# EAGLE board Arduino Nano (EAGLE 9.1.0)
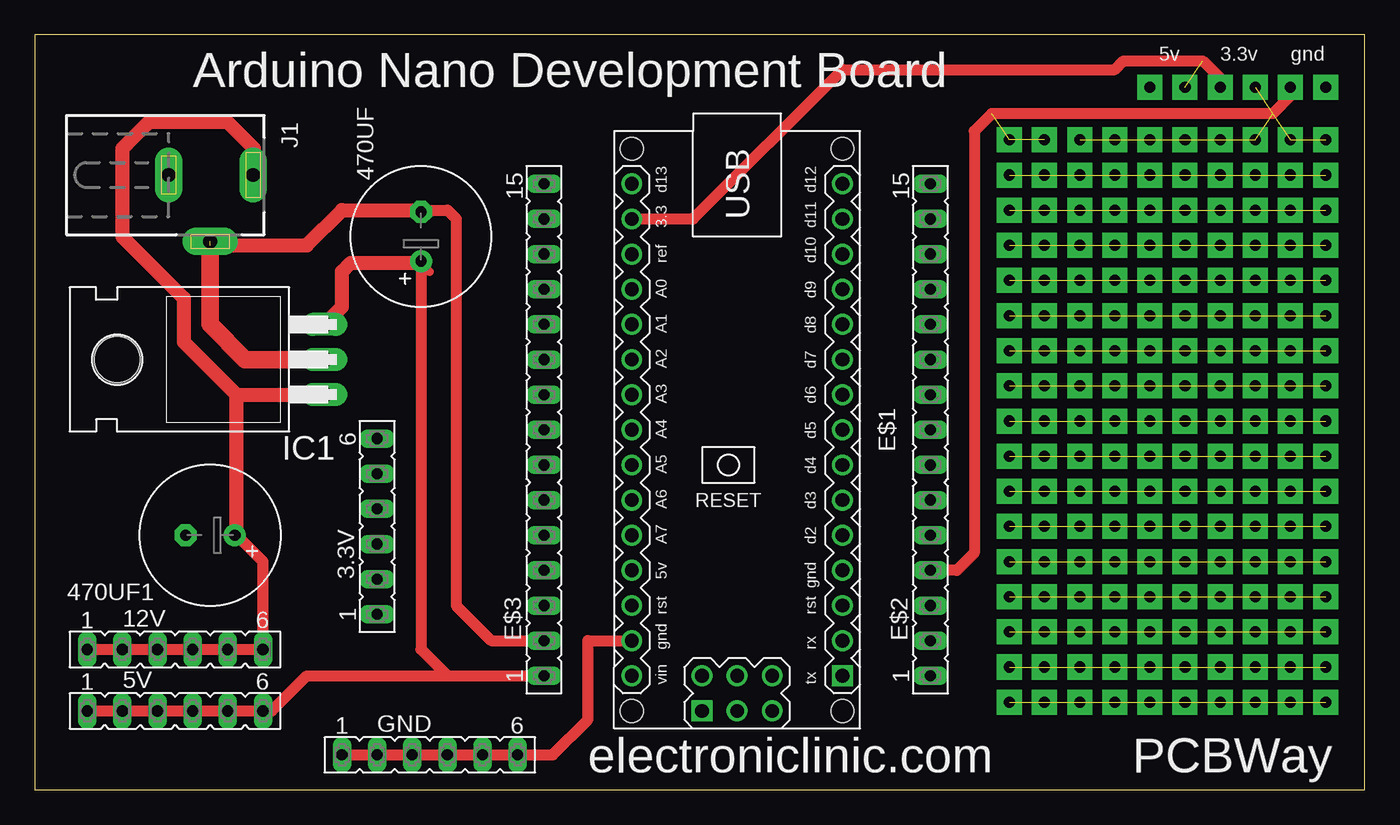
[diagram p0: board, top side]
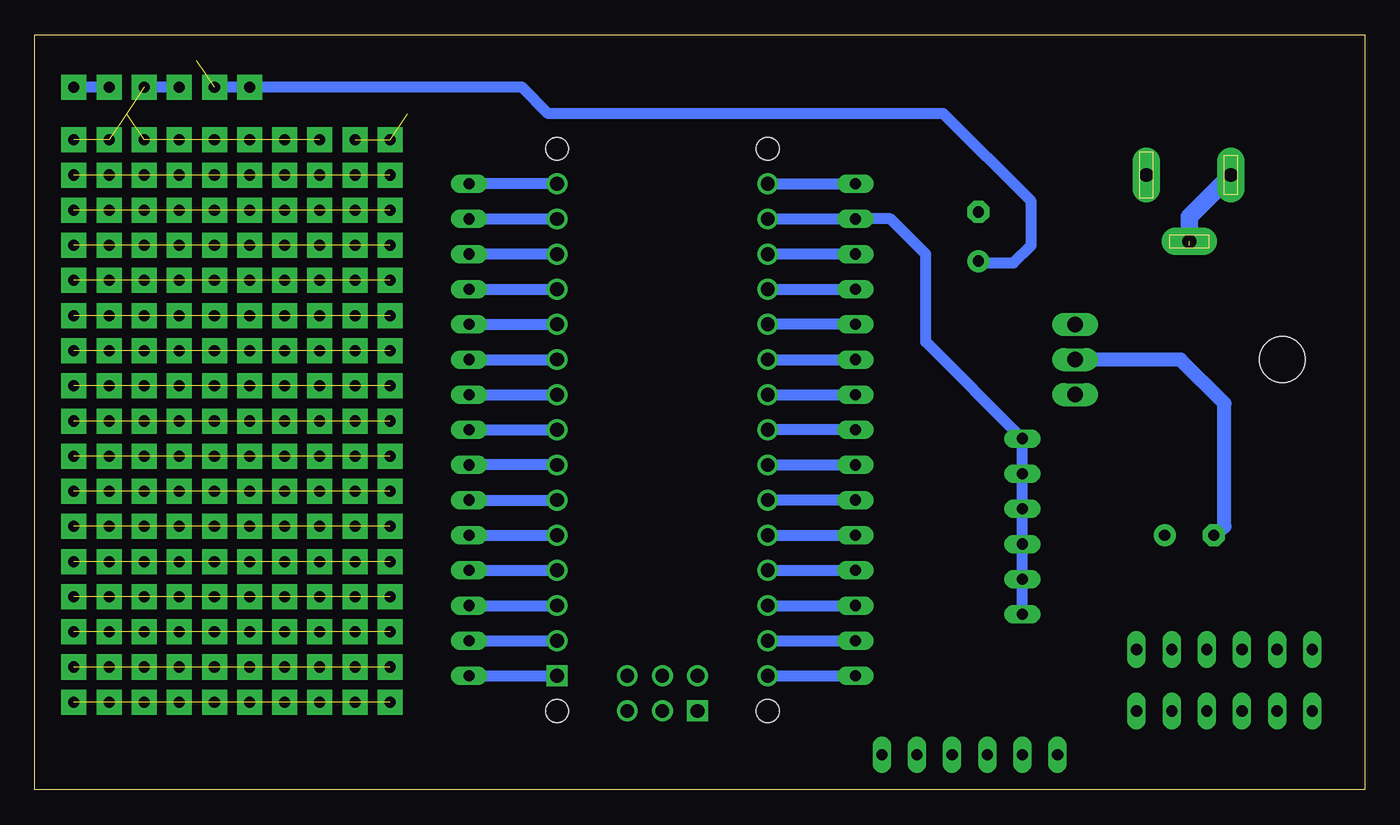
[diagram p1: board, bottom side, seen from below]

Size 96.19 x 54.6 mm. Coordinates in mm from the lower left corner, seen from the top.
Outline: 0,0 96.19,0 96.19,54.6 0,54.6 0,0
Copper layers (1*16): Top 0.035mm / dielectric 1.5mm / Bottom 0.035mm
Design rules "default": minimum track width 6mil, minimum drill 0.35mm, track to track 6mil, track to pad 6mil, pad to pad 6mil, via to via 6mil, smd to smd 6mil, copper to edge 40mil, drill to drill 6mil, minimum pad ring 10mil, minimum via ring 8mil, stop-mask expansion 4mil, vias tented up to drill 0mil, thermal gap 10mil

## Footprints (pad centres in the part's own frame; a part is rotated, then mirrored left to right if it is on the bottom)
FE06 = drill 0.813 long: 1 -6.35,0; 2 -3.81,0; 3 -1.27,0; 4 1.27,0; 5 3.81,0; 6 6.35,0
E3,5-10 = drill 0.813 pad 1.6: + -1.778,0 | drill 0.813 pad 1.6 octagon: - 1.778,0
ARDUINO-NANO-3.0#ISP = drill 1 square: J1.1 17.78,7.62; J4.1 20.32,-2.54 | drill 1: J1.2 15.24,7.62; J1.3 12.7,7.62; J1.4 10.16,7.62; J1.5 7.62,7.62; J1.6 5.08,7.62; J1.7 2.54,7.62; J1.8 0,7.62; J1.9 -2.54,7.62; J1.10 -5.08,7.62; J1.11 -7.62,7.62; J1.12 -10.16,7.62; J1.13 -12.7,7.62; J1.14 -15.24,7.62; J1.15 -17.78,7.62; J2.1 17.78,-7.62; J2.2 15.24,-7.62; J2.3 12.7,-7.62; J2.4 10.16,-7.62; J2.5 7.62,-7.62; J2.6 5.08,-7.62; J2.7 2.54,-7.62; J2.8 0,-7.62; J2.9 -2.54,-7.62; J2.10 -5.08,-7.62; J2.11 -7.62,-7.62; J2.12 -10.16,-7.62; J2.13 -12.7,-7.62; J2.14 -15.24,-7.62; J2.15 -17.78,-7.62; J4.2 17.78,-2.54; J4.3 20.32,0; J4.4 17.78,0; J4.5 20.32,2.54; J4.6 17.78,2.54 | hole 1.651: -20.32,7.62; -20.32,-7.62; 20.32,-7.62; 20.32,7.62
FE15 = drill 0.813 long: 1 -17.78,0; 2 -15.24,0; 3 -12.7,0; 4 -10.16,0; 5 -7.62,0; 6 -5.08,0; 7 -2.54,0; 8 0,0; 9 2.54,0; 10 5.08,0; 11 7.62,0; 12 10.16,0; 13 12.7,0; 14 15.24,0; 15 17.78,0
TO220H = drill 1.118 long: 1 -2.54,-10.16; 2 0,-10.16; 3 2.54,-10.16 | hole 3.302: 0,4.826
DCJ0202 = drill 1 pad 2 long: 1 0,3.1; 2 4.8,0; 3 0,-3

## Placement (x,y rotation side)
3.3V  [FE06]  24.77,19.05 90 top
5V  [FE06]  10.16,5.71 0 top
12V  [FE06]  10.16,10.16 0 top
470UF  [E3,5-10]  27.94,40.01 90 top
470UF1  [E3,5-10]  12.7,18.41 180 top
E$1  [ARDUINO-NANO-3.0#ISP]  50.8,26.04 270 top
E$2  [FE15]  64.77,26.04 90 top
E$3  [FE15]  36.83,26.04 90 top
GND  [FE06]  28.57,2.54 0 top
IC1  7805T  [TO220H]  10.79,31.11 90 top
J1  DCJ0202  [DCJ0202]  12.7,44.45 270 top

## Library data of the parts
3.3V 5V 12V E$2 E$3 GND = con-lsta
470UF 470UF1 = rcl
E$1 = diy-modules
IC1 = linear
J1 = con-jack; OC_FARNELL: unknown; OC_NEWARK: unknown

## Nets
5V: 5V.1 5V.2 5V.3 5V.4 5V.5 5V.6 E$1.J2.1 E$3.1 IC1.3
12V: 12V.1 12V.2 12V.3 12V.4 12V.5 12V.6 IC1.1
GND: E$1.J2.2 E$3.2 GND.1 GND.2 GND.4 GND.5 GND.6 IC1.2 J1.2 J1.3
S$2: E$1.J1.7 E$2.7
S$4: E$1.J1.15 E$2.15
S$5: E$1.J2.4 E$3.4
S$6: E$1.J1.14 E$2.14
S$7: E$1.J2.3 E$3.3
S$8: E$1.J1.13 E$2.13
S$9: E$1.J1.10 E$2.10
S$10: E$1.J1.12 E$2.12
S$11: 3.3V.1 3.3V.2 3.3V.3 3.3V.4 3.3V.5 3.3V.6 E$1.J1.4 E$1.J2.14 E$2.4 E$3.14
S$15: E$1.J1.9 E$2.9
S$16: E$1.J1.8 E$2.8
S$18: E$1.J1.3 E$2.3
S$19: E$1.J1.2 E$2.2
S$20: E$1.J1.1 E$2.1
S$21: E$1.J2.15 E$3.15
S$23: E$1.J2.13 E$3.13
S$24: E$1.J2.12 E$3.12
S$25: E$1.J2.11 E$3.11
S$26: E$1.J2.10 E$3.10
S$27: E$1.J2.9 E$3.9
S$28: E$1.J2.8 E$3.8
S$29: E$1.J2.7 E$3.7
S$30: E$1.J2.6 E$3.6
S$31: E$1.J2.5 E$3.5
S$32: E$1.J1.6 E$2.6
S$34: E$1.J1.5 E$2.5
S$38: E$1.J1.11 E$2.11

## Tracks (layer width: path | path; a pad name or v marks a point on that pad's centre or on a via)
5V
  Top 0.61: 28.57,37.47 27.94,38.1
  Top 0.813: 27.94,38.1 27.94,10.16 29.84,8.26 | 29.84,8.26 30.48,8.26 E$3.1 | 5V.1 5V.2 5V.3 5V.4 5V.5 5V.6 17.14,5.71 19.68,8.26 29.84,8.26
  Top 1.016: IC1.3 22.23,34.92 22.23,37.47 22.86,38.1 27.94,38.1
  Bottom 0.813: E$1.J2.1 E$3.1
12V
  Top 0.813: 12V.1 12V.2 12V.3 12V.4 12V.5 12V.6 16.51,16.51 14.61,18.41
  Top 1.016: 15.88,44.45 15.88,46.35 13.97,48.26 8.26,48.26 6.35,46.35 6.35,40.01 10.79,35.56 10.79,32.38 14.61,28.57 | 14.61,28.57 IC1.1 | 14.61,18.41 14.61,28.57
GND  (1 unrouted)
  Top 0.813: 27.94,41.91 29.84,41.91 30.48,41.27 30.48,13.34 33.02,10.79 E$3.2 | GND.1 GND.2 GND.4 GND.5 GND.6 37.47,2.54 40.01,5.08 40.01,10.79 E$1.J2.2
  Top 1.016: 12.7,39.37 19.68,39.37 22.23,41.91 27.94,41.91
  Top 1.27: 12.7,39.37 12.7,33.66 15.24,31.11 IC1.2
  Bottom 0.813: E$1.J2.2 E$3.2
  Bottom 1.016: 10.79,18.41 10.16,19.05 10.16,27.94 13.34,31.11 IC1.2
  Bottom 1.27: J1.3 12.7,41.45 J1.2
S$2
  Bottom 0.813: E$1.J1.7 E$2.7
S$4
  Bottom 0.813: E$1.J1.15 E$2.15
S$5
  Bottom 0.813: E$1.J2.4 E$3.4
S$6
  Bottom 0.813: E$2.14 E$1.J1.14
S$7
  Bottom 0.813: E$1.J2.3 E$3.3
S$8
  Bottom 0.813: E$1.J1.13 E$2.13
S$9
  Bottom 0.813: E$2.10 E$1.J1.10
S$10
  Bottom 0.813: E$2.12 E$1.J1.12
S$11  (via drill 0.8 pad 1.81)  (12 unrouted)
  Top 0.813: E$1.J2.14 47.62,41.27 58.42,52.07 78.11,52.07 78.74,52.7 84.45,52.7 85.72,51.44 v85.72,50.8 | v90.81,50.8 90.81,50.16 89.53,48.9 69.22,48.9 67.94,47.62 67.94,17.14 66.67,15.88 E$2.4
  Bottom 0.508: 27.94,38.1 26.04,38.1
  Bottom 0.813: 3.3V.1 3.3V.2 3.3V.3 3.3V.4 3.3V.5 3.3V.6 31.75,32.38 31.75,38.73 34.29,41.27 E$3.14 E$1.J2.14 | 27.94,38.1 25.4,38.1 24.13,39.37 24.13,42.55 30.48,48.9 59.05,48.9 60.96,50.8 v80.64,50.8 v83.19,50.8 | v85.72,50.8 v88.27,50.8 | v90.81,50.8 v93.34,50.8 | E$2.4 59.05,15.88 E$1.J1.4
  other vias: 70.48,46.99 73.03,46.99 75.56,46.99 78.11,46.99 80.64,46.99 83.19,46.99 85.72,46.99 88.27,46.99 90.81,46.99 93.34,46.99
S$13  (via drill 0.8 pad 1.81)  (9 unrouted)
  other vias: 70.48,44.45 73.03,44.45 75.56,44.45 78.11,44.45 80.64,44.45 83.19,44.45 85.72,44.45 88.27,44.45 90.81,44.45 93.34,44.45
S$14  (via drill 0.8 pad 1.81)  (9 unrouted)
  other vias: 70.48,41.91 73.03,41.91 75.56,41.91 78.11,41.91 80.64,41.91 83.19,41.91 85.72,41.91 88.27,41.91 90.81,41.91 93.34,41.91
S$15
  Bottom 0.813: E$2.9 E$1.J1.9
S$16
  Bottom 0.813: E$2.8 E$1.J1.8
S$18
  Bottom 0.813: E$2.3 E$1.J1.3
S$19
  Bottom 0.813: E$2.2 E$1.J1.2
S$20
  Bottom 0.813: E$2.1 E$1.J1.1
S$21
  Bottom 0.813: E$1.J2.15 E$3.15
S$22  (via drill 0.8 pad 1.81)  (9 unrouted)
  other vias: 70.48,39.37 73.03,39.37 75.56,39.37 78.11,39.37 80.64,39.37 83.19,39.37 85.72,39.37 88.27,39.37 90.81,39.37 93.34,39.37
S$23
  Bottom 0.813: E$3.13 E$1.J2.13
S$24
  Bottom 0.813: E$1.J2.12 E$3.12
S$25
  Bottom 0.813: E$3.11 E$1.J2.11
S$26
  Bottom 0.813: E$1.J2.10 E$3.10
S$27
  Bottom 0.813: E$1.J2.9 E$3.9
S$28
  Bottom 0.813: E$3.8 E$1.J2.8
S$29
  Bottom 0.813: E$1.J2.7 E$3.7
S$30
  Bottom 0.813: E$3.6 E$1.J2.6
S$31
  Bottom 0.813: E$1.J2.5 E$3.5
S$32
  Bottom 0.813: E$2.6 E$1.J1.6
S$34
  Bottom 0.813: E$2.5 E$1.J1.5
S$36  (via drill 0.8 pad 1.81)  (9 unrouted)
  other vias: 70.48,36.83 73.03,36.83 75.56,36.83 78.11,36.83 80.64,36.83 83.19,36.83 85.72,36.83 88.27,36.83 90.81,36.83 93.34,36.83
S$38
  Bottom 0.813: E$2.11 E$1.J1.11
S$39  (via drill 0.8 pad 1.81)  (9 unrouted)
  other vias: 70.48,34.29 73.03,34.29 75.56,34.29 78.11,34.29 80.64,34.29 83.19,34.29 85.72,34.29 88.27,34.29 90.81,34.29 93.34,34.29
S$40  (via drill 0.8 pad 1.81)  (9 unrouted)
  other vias: 70.48,31.75 73.03,31.75 75.56,31.75 78.11,31.75 80.64,31.75 83.19,31.75 85.72,31.75 88.27,31.75 90.81,31.75 93.34,31.75
S$41  (via drill 0.8 pad 1.81)  (9 unrouted)
  other vias: 70.48,29.21 73.03,29.21 75.56,29.21 78.11,29.21 80.64,29.21 83.19,29.21 85.72,29.21 88.27,29.21 90.81,29.21 93.34,29.21
S$42  (9 unrouted)
S$43  (9 unrouted)
S$44  (9 unrouted)
S$45  (via drill 0.8 pad 1.81)  (9 unrouted)
  other vias: 70.48,26.67 73.03,26.67 75.56,26.67 78.11,26.67 80.64,26.67 83.19,26.67 85.72,26.67 88.27,26.67 90.81,26.67 93.34,26.67
S$46  (via drill 0.8 pad 1.81)  (9 unrouted)
  other vias: 70.48,24.13 73.03,24.13 75.56,24.13 78.11,24.13 80.64,24.13 83.19,24.13 85.72,24.13 88.27,24.13 90.81,24.13 93.34,24.13
S$47  (via drill 0.8 pad 1.81)  (9 unrouted)
  other vias: 70.48,21.59 73.03,21.59 75.56,21.59 78.11,21.59 80.64,21.59 83.19,21.59 85.72,21.59 88.27,21.59 90.81,21.59 93.34,21.59
S$48  (via drill 0.8 pad 1.81)  (9 unrouted)
  other vias: 70.48,19.05 73.03,19.05 75.56,19.05 78.11,19.05 80.64,19.05 83.19,19.05 85.72,19.05 88.27,19.05 90.81,19.05 93.34,19.05
S$49  (via drill 0.8 pad 1.81)  (9 unrouted)
  other vias: 70.48,16.51 73.03,16.51 75.56,16.51 78.11,16.51 80.64,16.51 83.19,16.51 85.72,16.51 88.27,16.51 90.81,16.51 93.34,16.51
S$50  (via drill 0.8 pad 1.81)  (9 unrouted)
  other vias: 70.48,13.97 73.03,13.97 75.56,13.97 78.11,13.97 80.64,13.97 83.19,13.97 85.72,13.97 88.27,13.97 90.81,13.97 93.34,13.97
S$51  (via drill 0.8 pad 1.81)  (9 unrouted)
  other vias: 70.48,11.43 73.03,11.43 75.56,11.43 78.11,11.43 80.64,11.43 83.19,11.43 85.72,11.43 88.27,11.43 90.81,11.43 93.34,11.43
S$52  (via drill 0.8 pad 1.81)  (9 unrouted)
  other vias: 70.48,8.89 73.03,8.89 75.56,8.89 78.11,8.89 80.64,8.89 83.19,8.89 85.72,8.89 88.27,8.89 90.81,8.89 93.34,8.89
S$53  (via drill 0.8 pad 1.81)  (9 unrouted)
  other vias: 70.48,6.35 73.03,6.35 75.56,6.35 78.11,6.35 80.64,6.35 83.19,6.35 85.72,6.35 88.27,6.35 90.81,6.35 93.34,6.35

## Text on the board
tPlace: 5v | 3.3v | gnd | Arduino Nano Development Board | d13 | d12 | 3.3 | d11 | ref | d10 | A0 | d9 | A1 | d8 | A2 | d7 | A3 | d6 | A4 | d5 | A5 | d4 | A6 | d3 | A7 | d2 | 5v | gnd | rst | rst | gnd | rx | vin | tx | electroniclinic.com | PCBWay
